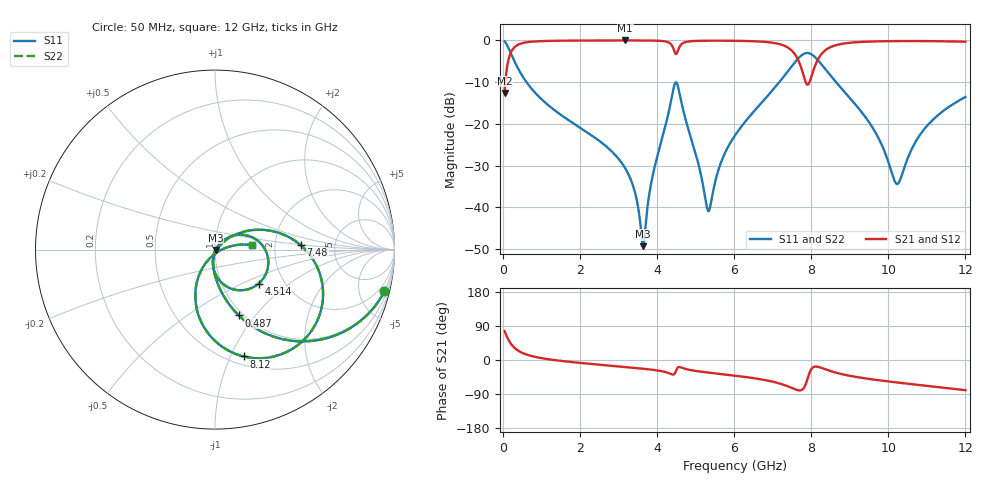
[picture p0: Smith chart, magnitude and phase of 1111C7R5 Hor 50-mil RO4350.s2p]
# GHz S MA R 50
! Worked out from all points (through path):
!   11951 points, 50 MHz to 12 GHz, reference 50 ohm
!   highest |S21| = -0.02 dB at 3.179 GHz (marker M1); lowest = -12.6 dB at 50 MHz (marker M2)
!   group delay of S21, straight-line fit = 20 ps
!   lowest |S11| = -49.3 dB at 3.643 GHz (marker M3), VSWR 1.01, Z = 50.3 - j0.158 ohm
!   |S11| at or under -10 dB: 617.6 MHz to 7.174 GHz (6.556 GHz wide, 168 % of centre); 8.646 GHz to end of sweep
!   |S22| runs from -49.3 to -0.2 dB; largest |S21 - S12| = 0
!   S11 on the Smith chart (normalised r, x): 50 MHz: 0.96, -8.12; 487 MHz: 0.96, -0.83; 4.514 GHz: 1.49, -0.62; 7.48 GHz: 2.83, +0.17; 8.12 GHz: 0.58, -1.12; 12 GHz: 1.52, +0.08
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0.05  0.9722 -13.9  0.234 76.1  0.234 76.1  0.9722 -13.9
0.204  0.713 -45.8  0.7008 44.2  0.7008 44.2  0.713 -45.8
0.487  0.3904 -70.1  0.92 19.9  0.92 19.9  0.3904 -70.1
2.042  0.08786 -97.2  0.9947 -8.0  0.9947 -8.0  0.08786 -97.2
3.179  0.02934 -104.4  0.9973 -18.5  0.9973 -18.5  0.02934 -104.4
3.433  0.015 -100.9  0.9971 -20.9  0.9971 -20.9  0.015 -100.9
3.643  0.003436 -27.1  0.9964 -23.0  0.9964 -23.0  0.003436 -27.1
4.034  0.04503 50.1  0.9895 -27.9  0.9895 -27.9  0.04503 50.1
4.367  0.1897 25.0  0.8966 -37.1  0.8966 -37.1  0.1897 25.0
4.514  0.3084 -37.9  0.6975 -24.1  0.6975 -24.1  0.3084 -37.9
4.705  0.1325 -89.6  0.9409 -22.4  0.9409 -22.4  0.1325 -89.6
5.328  0.009057 -35.1  0.9906 -33.1  0.9906 -33.1  0.009057 -35.1
6.025  0.07277 41.6  0.9881 -41.3  0.9881 -41.3  0.07277 41.6
7.48  0.4792 2.8  0.7673 -72.9  0.7673 -72.9  0.4792 2.8
7.771  0.6729 -27.6  0.4263 -78.1  0.4263 -78.1  0.6729 -27.6
8.017  0.6761 -62.3  0.3818 -22.4  0.3818 -22.4  0.6761 -62.3
8.12  0.6167 -74.9  0.5233 -17.2  0.5233 -17.2  0.6167 -74.9
8.599  0.3354 -108.1  0.8634 -32.2  0.8634 -32.2  0.3354 -108.1
10.009  0.0342 -109.3  0.9784 -56.7  0.9784 -56.7  0.0342 -109.3
10.254  0.01929 -47.4  0.9807 -59.7  0.9807 -59.7  0.01929 -47.4
10.915  0.08438 11.9  0.9802 -67.3  0.9802 -67.3  0.08438 11.9
12  0.21 6.7  0.9634 -79.6  0.9634 -79.6  0.21 6.7
